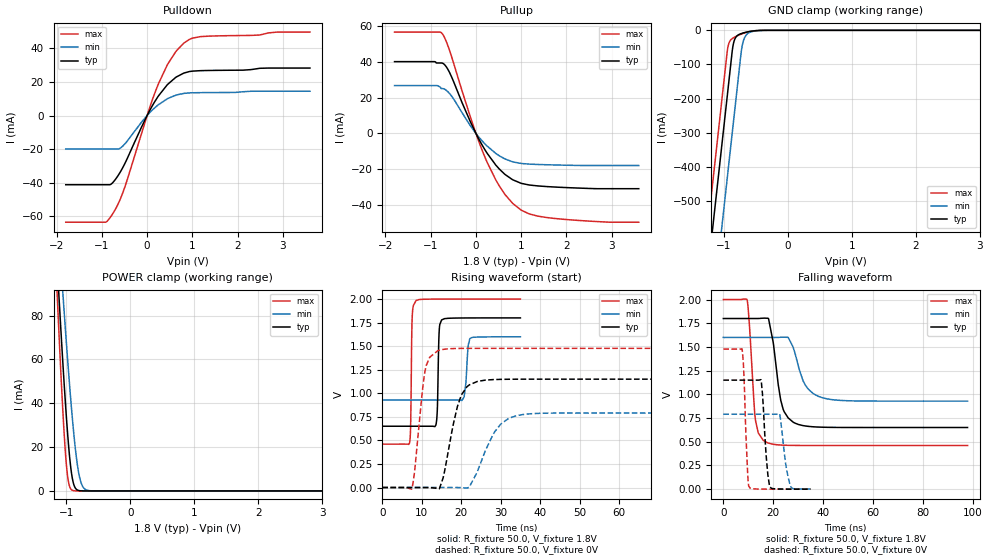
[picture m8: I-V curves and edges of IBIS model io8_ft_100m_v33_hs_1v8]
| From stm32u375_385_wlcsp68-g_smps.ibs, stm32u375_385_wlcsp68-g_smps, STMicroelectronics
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[Model]   io8_ft_100m_v33_hs_1v8
Model_type I/O
Polarity   Non-Inverting
Enable   Active-Low
| CAP_THRESHOLD on pad IOFT is "UDTCAPC" :
| Rising=30.0% of vddiom   Falling=70.0% of vddiom
| C_comp min and max val. don't necessarily correlate with the min and max pvt
| but are the smallest and greatest pad capacitance found.
| var   typ   min   max
C_comp   4.46110pF  4.37696pF  4.58318pF
|C_comp_pullup   2.75073pF  2.57455pF  2.90964pF
|C_comp_pulldown   1.71037pF  1.80241pF  1.67354pF
Vinl = 800.0mV
Vinh = 1.0V
Vmeas = 900.0mV   | Reference voltage for timing measurements
Cref  = 50.0pF   | Timing specification test load capacitance value
Rref  = 1.0MOhm   | Timing specification test load resistance value
Vref  = 990.0mV   | Timing specification test load voltage
[Model Spec]
| TIME_THRESHOLD on pin ZIV33M is "CMOS" :
| Rising=50.0% of vddiom   Falling=50.0% of vddiom
Vinl 689.50000mV 614.50000mV 772.50000mV
Vinh 1.08250V 955.50000mV 1.18750V
| variable   typ   min   max
[Temperature Range] 25.0 130.0 -40.0
| variable   typ   min   max
[Voltage Range] 1.8V 1.6V 2.0V
| variable   typ   min   max
[POWER Clamp Reference] 1.8V 1.6V 2.0V
| variable   typ   min   max
[GND Clamp Reference] 0V 0V 0V
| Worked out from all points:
|   slope of the pulldown table from 0 to 0.27 V, typ, clamps not added: 21.9 ohm
|   slope of the pullup table from 0 to 0.27 V, typ, clamps not added: 22.8 ohm
|   GND clamp passes 1 mA (typ) near -0.50 V on its own axis
|   POWER clamp passes 1 mA (typ) near -0.85 V on its own axis
|   rising waveform, R_fixture 50.0, V_fixture 1.8V: 20-80 % time 341ps typ, 646ps min, 269ps max; typ from 0.65 V to 1.8 V
|   falling waveform, R_fixture 50.0, V_fixture 1.8V: 20-80 % time 3.77ns typ, 5.46ns min, 2.15ns max; typ from 1.8 V to 0.65 V
|   rising waveform, R_fixture 50.0, V_fixture 0V: 20-80 % time 3.48ns typ, 5.28ns min, 2.14ns max; typ from 0 V to 1.15 V
|   falling waveform, R_fixture 50.0, V_fixture 0V: 20-80 % time 1.68ns typ, 2.35ns min, 1.25ns max; typ from 1.15 V to 0 V
[POWER Clamp]
-1.8V     478.8mA    439.5mA    561.1mA
-1.14V    101.7mA    127.5mA    87.74mA
-1.11V    86.11mA    114.3mA    68.77mA
-1.05V    56.42mA    88.49mA    34.19mA
-1.01V    38.33mA    71.95mA    15.91mA
-970mV    22.56mA    56.16mA    4.74mA
-910mV    6.426mA    34.56mA    354.8uA
-850mV    950.4uA    17.03mA    20.6uA
-800mV    153.4uA    7.248mA    1.891uA
-750mV    23.75uA    2.361mA    173.6nA
-670mV    1.188uA    286.7uA    3.927nA
3.6V      0A         0A         0A
[GND Clamp]
-1.8V     -1.641A    -1.882A    -1.509A
-1.24V    -689.3mA   -929.9mA   -557.3mA
-1.05V    -366.3mA   -606.9mA   -234.3mA
-950mV    -196.3mA   -436.9mA   -64.35mA
-930mV    -162.3mA   -402.9mA   -42.64mA
-870mV    -60.33mA   -300.9mA   -24.14mA
-850mV    -37.9mA    -266.9mA   -21.7mA
-770mV    -12.83mA   -130.9mA   -14.29mA
-730mV    -9.517mA   -63.9mA    -11.18mA
-690mV    -7.204mA   -27.69mA   -8.428mA
-530mV    -1.58mA    -2.534mA   -1.415mA
3.6V      1.308nA    187.1nA    582.2pA
| variable   typ   min   max
[Pullup Reference] 1.8V 1.6V 2.0V
| variable   typ   min   max
[Pulldown Reference] 0V 0V 0V
[Pullup]
-1.8V     40.03mA    26.7mA     56.51mA
-870mV    39.28mA    26.7mA     56.51mA
-740mV    39.18mA    25mA       55.44mA
-590mV    34.28mA    22.43mA    46.72mA
-120mV    6.328mA    4.158mA    8.961mA
250mV     -11.14mA   -7.108mA   -16.23mA
440mV     -17.67mA   -11.15mA   -25.97mA
630mV     -22.57mA   -14.06mA   -33.59mA
1V        -27.82mA   -16.74mA   -42.77mA
1.37V     -29.26mA   -17.3mA    -46.1mA
1.74V     -29.87mA   -17.57mA   -47.39mA
3.6V      -30.8mA    -17.88mA   -49.48mA
[Pulldown]
-1.8V     -41.16mA   -19.96mA   -63.43mA
-920mV    -41.16mA   -19.96mA   -63.43mA
-780mV    -40.43mA   -19.96mA   -59.18mA
-620mV    -34.74mA   -19.77mA   -51.3mA
-510mV    -29.46mA   -17.38mA   -43.8mA
0V        155.1fA    35.29pA    0A
250mV     11.64mA    6.428mA    18.87mA
460mV     18.67mA    10.12mA    30.76mA
630mV     22.61mA    12.05mA    37.86mA
810mV     25.21mA    13.14mA    43.03mA
1.18V     26.67mA    13.59mA    46.9mA
3.6V      28.21mA    14.43mA    49.6mA
[Ramp]
dV/dt_r 690.02397mV/3.41535ns 474.37403mV/5.17708ns 886.36631mV/2.12868ns
dV/dt_f 689.75464mV/3.63921ns 402.89509mV/5.41563ns 923.68058mV/2.14732ns
R_load = 50.0
| Removed startup time: 0s 0s 0s  .
| Removed end time: 34.95ns.
[Rising Waveform]
R_fixture   = 50.0
V_fixture   = 1.8V
V_fixture_min = 1.6V
V_fixture_max = 2.0V
0s        650.4mV    928.3mV    460.5mV
6.9ns     650.4mV    928.3mV    476.4mV
7.15ns    650.4mV    928.3mV    628.6mV
7.55ns    650.4mV    928.3mV    1.795V
8.55ns    650.4mV    928.3mV    1.985V
13.55ns   662.2mV    928.3mV    2V
15ns      1.778V     928.3mV    2V
20.7ns    1.799V     961.3mV    2V
22.15ns   1.8V       1.581V     2V
34.95ns   1.8V       1.6V       2V
| Removed startup time: 0s 0s 0s  .
| Removed end time: 97.95ns.
[Falling Waveform]
R_fixture   = 50.0
V_fixture   = 1.8V
V_fixture_min = 1.6V
V_fixture_max = 2.0V
0s        1.8V       1.6V       2V
9.5ns     1.8V       1.6V       1.999V
12.85ns   1.8V       1.6V       735.3mV
16.5ns    1.804V     1.6V       505.6mV
18.15ns   1.795V     1.6V       485.1mV
24ns      841.8mV    1.603V     464.1mV
28ns      706.6mV    1.497V     461.5mV
32.9ns    666.6mV    1.097V     460.7mV
40ns      653.3mV    962.2mV    460.6mV
97.95ns   650.4mV    928.5mV    460.5mV
| Removed startup time: 0s 0s 0s  .
| Removed end time: 97.9ns.
[Rising Waveform]
R_fixture   = 50.0
V_fixture   = 0V
V_fixture_min = 0V
V_fixture_max = 0V
0s        5.001nV    122.3nV    3.682nV
7.45ns    4.454nV    122.2nV    -15.81mV
10.85ns   509.5nV    121.8nV    1.245V
14ns      -9.612mV   118.7nV    1.451V
15.4ns    104.4mV    123.2nV    1.466V
20ns      982.2mV    -433.9uV   1.476V
24ns      1.125V     162.7mV    1.477V
28.45ns   1.146V     591.5mV    1.477V
34ns      1.15V      763.1mV    1.477V
97.9ns    1.15V      790.6mV    1.477V
| Removed startup time: 0s 0s 0s  .
| Removed end time: 34.95ns.
[Falling Waveform]
R_fixture   = 50.0
V_fixture   = 0V
V_fixture_min = 0V
V_fixture_max = 0V
0s        1.15V      790.6mV    1.477V
7.5ns     1.15V      790.6mV    1.478V
8.15ns    1.15V      790.6mV    1.263V
9.8ns     1.15V      790.6mV    145.7mV
10.7ns    1.15V      790.6mV    10.51mV
15.15ns   1.148V     790.6mV    879.3uV
18.55ns   27.86mV    790.6mV    244.7uV
22.6ns    1.762mV    789mV      59.43uV
27.15ns   444.8uV    20.91mV    12.75uV
34.95ns   103.2uV    2.032mV    962.8nV
